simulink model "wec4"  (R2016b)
settings: Solver=ode4  StartTime=0  StopTime=1000  FixedStep=0.005  MaxStep=0.005  RelTol=1e-3  EnableMultiTasking=on
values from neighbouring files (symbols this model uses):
  arAdaptiveLawData = 1/2*zModelSimple.zModelPto.arFreq.*     zModelSimple.zModelPto.arMagnitude./     cos(zModelSimple.zModelPto.arPhase*pi/180+pi/2)    [IMPACT_Control.m]
  arAdaptiveLawDataX = 1/2*zModelSimpleX.zModelPto.arFreq.*         zModelSimpleX.zModelPto.arMagnitude./         cos(zModelSimpleX.zModelPto.arPhase*pi/180+pi/2)    [IMPACT_Control.m]
  arControllerRampGain = [0,0,1,1]    [IMPACT_Control.m]
  arControllerRampTime = [0 rStartRampTime rStartRampTime+rRampTimeLength 8000]    [IMPACT_Control.m]
  arEkfInitialisation = zeros(1,11)    [IMPACT_Control.m]
  arEkfInitialisationX = zeros(1,11)    [IMPACT_Control.m]
  arFrequency = zModelSimple.zModelPto.arFreq    [IMPACT_Control.m]
  arFrequencyRange = zModelSimple.zModelPto.arFreq    [IMPACT_Control.m]
  arFrequencyX = zModelSimpleX.zModelPto.arFreq    [IMPACT_Control.m]
  arImpedance = 1./zModelSimple.zModelPto.arMagnitude./zModelSimple.zModelPto.arFreq    [IMPACT_Control.m]
  arImpedanceX = 1./zModelSimpleX.zModelPto.arMagnitude./zModelSimpleX.zModelPto.arFreq    [IMPACT_Control.m]
  CentralPTOPreload = -1.6113e+07    (= -16113000)    [wecSimInputFile.m]
  F1 = [4.243 2.375 -12.243]    [wecSimInputFile.m]
  F2 = [4.243 -2.375 -12.243]    [wecSimInputFile.m]
  F3 = [-4.243 -2.375 -12.243]    [wecSimInputFile.m]
  F4 = [-4.243 2.375 -12.243]    [wecSimInputFile.m]
  FC = [0 0 -14]    [wecSimInputFile.m]
  iAdaptiveDamping = 0    [wec4IMPACT_Project.m]    (also in IMPACT_Control.m = handles.iAdaptiveDamping; wec1_IMPACT_Project.m; wec2_IMPACT_Project.m; wec3_IMPACT_Project.m)
  iControlType = 2    [wec4IMPACT_Project.m]    (also in IMPACT_Control.m = handles.iControlType; wec1_IMPACT_Project.m = 1; wec2_IMPACT_Project.m = 1; wec3_IMPACT_Project.m = 1)
  iPtoPositionConstraint = 1    [wec4IMPACT_Project.m]    (also in IMPACT_Control.m = handles.iPtoPositionConstraint; wec1_IMPACT_Project.m = 0; wec2_IMPACT_Project.m; wec3_IMPACT_Project.m)
  iSensorNoise = 0    [IMPACT_Control.m]
  m = m+1    (= 2)    [checkParamFile.m]
  PTOrotation = atan((T1(2)-F1(2))/(T1(1)-F1(1)))    [wecSimInputFile.m]
  rCogFloater = -8    [wec4_IMPACT_Model.m]    (also in paramInitial.m = get( handles.edit_rCogFloater, 'String' ); wec1_IMPACT_Model.m = -18; wec2_IMPACT_Model.m = -8.5; wec3_IMPACT_Model.m = -0.7)
  rCogSpar = -36.6    [wec4_IMPACT_Model.m]    (also in paramInitial.m = get( handles.edit_rCogSpar, 'String' ); wec3_IMPACT_Model.m = -21.3; wec3_IMPACT_Model2.m = -21.3)
  rDisplacementLimit = 10.000000    (= 10)    [wec4IMPACT_Project.m]    (also in IMPACT_Control.m = getValue(handles.edit_displacementLimit); wec1_IMPACT_Project.m; wec2_IMPACT_Project.m; wec3_IMPACT_Project.m = 3)
  rDisplacementLimitX = 10.000000    (= 10)    [wec4IMPACT_Project.m]    (also in IMPACT_Control.m = getValue(handles.edit_displacementLimitX); wec1_IMPACT_Project.m = 0; wec2_IMPACT_Project.m; wec3_IMPACT_Project.m = 0)
  rGainForAntiWIndUp = tfControllerDiscrete.rGain    [IMPACT_Control.m]
  rGainForAntiWIndUpX = tfControllerXDiscrete.rGain    [IMPACT_Control.m]
  rMaxForcePto = 300000000.000000    (= 300000000)    [wec4IMPACT_Project.m]    (also in IMPACT_Control.m = getValue(handles.edit_maxForcePto); wec1_IMPACT_Project.m = 1e+15; wec2_IMPACT_Project.m = 1e+15; wec3_IMPACT_Project.m = 1000000000)
  rMinForcePto = -300000000.000000    (= -300000000)    [wec4IMPACT_Project.m]    (also in IMPACT_Control.m = getValue(handles.edit_minForcePto); wec1_IMPACT_Project.m = -1e+15; wec2_IMPACT_Project.m = -1e+15; wec3_IMPACT_Project.m = -1000000000)
  rMooringX = 20000    [wec4_IMPACT_Model.m]    (also in paramInitial.m = get( handles.edit_rMooringX, 'String' ); wec3_IMPACT_Model.m = 10000; wec3_IMPACT_Model2.m = 10000)
  rMooringZ = 10000    [wec4_IMPACT_Model.m]    (also in paramInitial.m = get( handles.edit_rMooringZ, 'String' ); wec3_IMPACT_Model.m = 0; wec3_IMPACT_Model2.m = 0)
  rOutputSampleTime = 0.010000    (= 0.01)    [wec4IMPACT_Project.m]    (also in IMPACT_Control.m = getValue(handles.edit_outputSampleTime); wec1_IMPACT_Project.m; wec2_IMPACT_Project.m; wec3_IMPACT_Project.m)
  rPassiveDampingGain = -604830.000000    (= -604830)    [wec4IMPACT_Project.m]    (also in IMPACT_Control.m = getValue(handles.edit_gainPLD); wec1_IMPACT_Project.m = -214018.1537; wec2_IMPACT_Project.m = -1948070; wec3_IMPACT_Project.m = -519390)
  rPassiveDampingGainX = -278660.000000    (= -278660)    [wec4IMPACT_Project.m]    (also in IMPACT_Control.m = getValue(handles.edit_gainPLDX); wec1_IMPACT_Project.m = 0; wec2_IMPACT_Project.m = 0; wec3_IMPACT_Project.m = 0)
  rTetherPretension = 1.6113e+07    (= 16113000)    [wec4_IMPACT_Model.m]    (also in paramInitial.m = get( handles.edit_rTetherPretension, 'String' ); wec3_IMPACT_Model.m = 0; wec3_IMPACT_Model2.m = 0)
  rTetherSpring = 500000    [wec4_IMPACT_Model.m]    (also in paramInitial.m = get( handles.edit_rTetherSpring, 'String' ); wec3_IMPACT_Model.m = 0; wec3_IMPACT_Model2.m = 0)
  rUpperFrequencyLimit = EKFFloater.upperFreq    [IMPACT_Control.m]
  rXf = 4.243    [wec4AdditionalParams.m]
  rXs = 16.075    [wec4AdditionalParams.m]
  rYf = 2.375    [wec4AdditionalParams.m]
  rYs = 16.075    [wec4AdditionalParams.m]
  rZf = 4.243    [wec4AdditionalParams.m]
  rZs = 2.4350    (= 2.435)    [wec4AdditionalParams.m]
  rZTetherF = 6    [wec4AdditionalParams.m]
  rZTetherS = 2.4350    (= 2.435)    [wec4AdditionalParams.m]
  s = tf('s')    [wec4_IMPACT_Model.m]    (also in IMPACT_Control.m; wec1_IMPACT_Model.m; wec2_IMPACT_Model.m; wec3_IMPACT_Model.m)
  SidePTO1Preload = PreloadPTOCorner    (= 0)    [wecSimInputFile.m]
  SidePTO2Preload = PreloadPTOCorner    (= 0)    [wecSimInputFile.m]
  SidePTO3Preload = PreloadPTOCorner    (= 0)    [wecSimInputFile.m]
  SidePTO4Preload = PreloadPTOCorner    (= 0)    [wecSimInputFile.m]
  simu = simulationClass()    [wecSimInputFile.m]
  T1 = [16.075 16.075 -34.165]    [wecSimInputFile.m]
  T2 = [16.075 -16.075 -34.165]    [wecSimInputFile.m]
  T3 = [-16.075 -16.075 -34.165]    [wecSimInputFile.m]
  T4 = [-16.075 16.075 -34.165]    [wecSimInputFile.m]
  TC = [0 0 -34.165]    [wecSimInputFile.m]
  waves = waveClass('irregular')    [wecSimInputFile.m]
  Z = magPhaseToComplex(zModelTf)    [IMPACT_Control.m]
undefined symbols (not defined in the file or in its folder): arControllerDiscreteDen, arControllerDiscreteNum, arControllerDiscreteXDen, arControllerDiscreteXNum, arExcForceFloaterDen, arExcForceFloaterNum, arExcForceFloaterXDen, arExcForceFloaterXNum, arExcForceSparDen, arExcForceSparNum, arExcForceSparXDen, arExcForceSparXNum, arFexcFloaterDen, arFexcFloaterNum, arFexcFloaterXDen, arFexcFloaterXNum, arFexcSparDen, arFexcSparNum, arFexcSparXDen, arFexcSparXNum, Body, body, constraint, CTTime, deg, Elements, geometry, IRKB, kg, lenJ, mooring, N, pto, rAccelerationGainFloater, rAccelerationGainFloaterX, rAccelerationGainSpar, rAccelerationGainSparX, rad, rBuoyancyGainFloater, rBuoyancyGainFloaterX, rBuoyancyGainSpar, rBuoyancyGainSparX, rDampingGainFloater, rDampingGainFloaterX, rDampingGainSpar, rDampingGainSparX, Rigid, rMaxFocePto, wec4_float, wec4_reactor, WECSim_Lib, X, Y
libraries: nesl_utility x380, sm_lib x170, vrlib x91, simulink x12, WECSim_Lib x4
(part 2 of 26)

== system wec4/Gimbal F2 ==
  Assignment : Assignment  DiagnosticForDimensions=Warning  IndexOptions=Index vector (dialog)  Indices=[4 5 6]  OutputSizes=1
  Assignment1 : Assignment  DiagnosticForDimensions=Warning  IndexOptions=Index vector (dialog)  Indices=[4 5 6]  OutputSizes=1
  Assignment2 : Assignment  DiagnosticForDimensions=Warning  IndexOptions=Index vector (dialog)  Indices=[4 5 6]  OutputSizes=1
  Assignment3 : Assignment  DiagnosticForDimensions=Warning  IndexOptions=Index vector (dialog)  Indices=2  OutputSizes=1
  Assignment4 : Assignment  DiagnosticForDimensions=Warning  IndexOptions=Index vector (dialog)  Indices=2  OutputSizes=1
  CONSTRAINT (Gimbal Joint) : sm_lib/Joints/Gimbal Joint  SenseConstraintForce=on  SenseConstraintForceX=off  SenseConstraintForceY=off  SenseConstraintForceZ=off  SenseConstraintTorque=on  SenseConstraintTorqueX=off  SenseConstraintTorqueY=off  SenseConstraintTorqueZ=off  SenseTotalForce=off  SenseTotalForceX=off  SenseTotalForceY=off  SenseTotalForceZ=off  SenseTotalTorque=off  SenseTotalTorqueX=off  SenseTotalTorqueY=off  SenseTotalTorqueZ=off  CompositeWrenchDir=BaseOnFollower  CompositeWrenchFrame=BaseFrame  RxEquilibriumPosition=0  RxEquilibriumPositionUnits=rad  RxSpringStiffness=top_const_k  RxSpringStiffnessUnits=N*m/rad  RxDampingCoefficient=top_const_c  RxDampingCoefficientUnits=N*m/(rad/s)  RxTorqueActuationMode=NoTorque  RxMotionActuationMode=ComputedMotion  RxSensePosition=on  RxSenseVelocity=on  RxSenseAcceleration=on  RxSenseTorqueForce=off  RxPositionTargetSpecify=off  RxPositionTargetPriority=High  RxPositionTargetValue=0  RxPositionTargetValueUnits=deg  RxVelocityTargetSpecify=off  RxVelocityTargetPriority=High  RxVelocityTargetValue=0  RxVelocityTargetValueUnits=deg/s  RyEquilibriumPosition=0  RyEquilibriumPositionUnits=rad  RySpringStiffness=top_const_k  RySpringStiffnessUnits=N*m/rad  RyDampingCoefficient=top_const_c  RyDampingCoefficientUnits=N*m/(rad/s)  RyTorqueActuationMode=NoTorque  RyMotionActuationMode=ComputedMotion  RySensePosition=on  RySenseVelocity=on  RySenseAcceleration=on  RySenseTorqueForce=off  RyPositionTargetSpecify=off  RyPositionTargetPriority=High  RyPositionTargetValue=0  RyPositionTargetValueUnits=deg  RyVelocityTargetSpecify=off  RyVelocityTargetPriority=High  RyVelocityTargetValue=0  RyVelocityTargetValueUnits=deg/s  RzEquilibriumPosition=0  RzEquilibriumPositionUnits=rad  RzSpringStiffness=top_const_k  RzSpringStiffnessUnits=N*m/rad  RzDampingCoefficient=top_const_c  RzDampingCoefficientUnits=N*m/(rad/s)  RzTorqueActuationMode=NoTorque  RzMotionActuationMode=ComputedMotion  RzSensePosition=on  RzSenseVelocity=on  RzSenseAcceleration=on  RzSenseTorqueForce=off  RzPositionTargetSpecify=off  RzPositionTargetPriority=High  RzPositionTargetValue=0  RzPositionTargetValueUnits=deg  RzVelocityTargetSpecify=off  RzVelocityTargetPriority=High  RzVelocityTargetValue=0  RzVelocityTargetValueUnits=deg/s
  Constant : Constant  Value=[0 0 0 0 0 0]
  Constant1 : Constant  Value=[0 0 0 0 0 0]
  Constant2 : Constant  Value=[0 0 0 0 0 0]
  Gain{1..5} (5 alike) : Gain  Gain=-1
  Mux : Mux  Inputs=2
  Mux1 : Mux
  Mux2 : Mux  Inputs=3
  Mux3 : Mux  Inputs=3
  Mux4 : Mux  Inputs=3
  PS-Simulink Converter{1..11} (11 alike) : nesl_utility/PS-Simulink Converter  PhysicalDomain=network_engine_domain  SubClassName=ps_output  LeftPortType=input  RightPortType=output  PseudoPeriodic=off  Frequencies=[]  Unit=1  AffineConversion=off
  Rigid Transform (Position) : sm_lib/Frames and Transforms/Rigid Transform  TranslationMethod=Cartesian  TranslationStandardOffset=0  TranslationLengthUnit=m  TranslationStandardAxis=+Z  TranslationCartesianOffset=constraint.initDisp.initLinDisp+constraint.loc  TranslationROffset=0  TranslationROffsetUnits=m  TranslationZOffset=0  TranslationZOffsetUnits=m  TranslationThetaOffset=0  TranslationThetaOffsetUnits=deg  RotationMethod=None  RotationAngleUnits=rad  RotationStandardAxis=+Y  RotationAngle=0  RotationArbitraryAxis=[0 1 0]  FollAlignAxisA=+X  BaseAlignAxisA=+Y  FollAlignAxisB=+Y  BaseAlignAxisB=+Z  RotationSequenceAxes=FollowerAxes  RotationSequence=XYX  RotationSequenceAngles=[0 0 0]  RotationSequenceAnglesUnits=deg  RotationMatrix=[1 0 0; 0 1 0; 0 0 1]
  Rigid Transform (Position)1 : sm_lib/Frames and Transforms/Rigid Transform  TranslationMethod=Cartesian  TranslationStandardOffset=0  TranslationLengthUnit=m  TranslationStandardAxis=+Z  TranslationCartesianOffset=constraint.initDisp.initLinDisp+constraint.loc  TranslationROffset=0  TranslationROffsetUnits=m  TranslationZOffset=0  TranslationZOffsetUnits=m  TranslationThetaOffset=0  TranslationThetaOffsetUnits=deg  RotationMethod=None  RotationAngleUnits=rad  RotationStandardAxis=+Y  RotationAngle=0  RotationArbitraryAxis=[0 1 0]  FollAlignAxisA=+X  BaseAlignAxisA=+Y  FollAlignAxisB=+Y  BaseAlignAxisB=+Z  RotationSequenceAxes=FollowerAxes  RotationSequence=XYX  RotationSequenceAngles=[0 0 0]  RotationSequenceAnglesUnits=deg  RotationMatrix=[1 0 0; 0 1 0; 0 0 1]
  Rigid Transform (90 X) : sm_lib/Frames and Transforms/Rigid Transform  TranslationMethod=None  TranslationStandardOffset=0  TranslationLengthUnit=m  TranslationStandardAxis=+Z  TranslationCartesianOffset=constraint.loc  TranslationROffset=0  TranslationROffsetUnits=m  TranslationZOffset=0  TranslationZOffsetUnits=m  TranslationThetaOffset=0  TranslationThetaOffsetUnits=deg  RotationMethod=StandardAxis  RotationAngleUnits=deg  RotationStandardAxis=+X  RotationAngle=90  RotationArbitraryAxis=[0 1 0]  FollAlignAxisA=+X  BaseAlignAxisA=+Y  FollAlignAxisB=+Y  BaseAlignAxisB=+Z  RotationSequenceAxes=FollowerAxes  RotationSequence=XYX  RotationSequenceAngles=[0 0 0]  RotationSequenceAnglesUnits=deg  RotationMatrix=[1 0 0; 0 1 0; 0 0 1]
  Rigid Transform (90 X)1 : sm_lib/Frames and Transforms/Rigid Transform  TranslationMethod=None  TranslationStandardOffset=0  TranslationLengthUnit=m  TranslationStandardAxis=+Z  TranslationCartesianOffset=constraint.loc  TranslationROffset=0  TranslationROffsetUnits=m  TranslationZOffset=0  TranslationZOffsetUnits=m  TranslationThetaOffset=0  TranslationThetaOffsetUnits=deg  RotationMethod=StandardAxis  RotationAngleUnits=deg  RotationStandardAxis=+X  RotationAngle=90  RotationArbitraryAxis=[0 1 0]  FollAlignAxisA=+X  BaseAlignAxisA=+Y  FollAlignAxisB=+Y  BaseAlignAxisB=+Z  RotationSequenceAxes=FollowerAxes  RotationSequence=XYX  RotationSequenceAngles=[0 0 0]  RotationSequenceAnglesUnits=deg  RotationMatrix=[1 0 0; 0 1 0; 0 0 1]
  Rigid Transform (Orientation) : sm_lib/Frames and Transforms/Rigid Transform  TranslationMethod=None  TranslationStandardOffset=0  TranslationLengthUnit=m  TranslationStandardAxis=+Z  TranslationCartesianOffset=constraint.loc  TranslationROffset=0  TranslationROffsetUnits=m  TranslationZOffset=0  TranslationZOffsetUnits=m  TranslationThetaOffset=0  TranslationThetaOffsetUnits=deg  RotationMethod=RotationMatrix  RotationAngleUnits=rad  RotationStandardAxis=+Y  RotationAngle=0  RotationArbitraryAxis=[0 1 0]  FollAlignAxisA=+X  BaseAlignAxisA=+Y  FollAlignAxisB=+Y  BaseAlignAxisB=+Z  RotationSequenceAxes=FollowerAxes  RotationSequence=XYX  RotationSequenceAngles=[0 0 0]  RotationSequenceAnglesUnits=deg  RotationMatrix=constraint.orientation.rotationMatrix
  Rigid Transform (Orientation)1 : sm_lib/Frames and Transforms/Rigid Transform  TranslationMethod=None  TranslationStandardOffset=0  TranslationLengthUnit=m  TranslationStandardAxis=+Z  TranslationCartesianOffset=constraint.loc  TranslationROffset=0  TranslationROffsetUnits=m  TranslationZOffset=0  TranslationZOffsetUnits=m  TranslationThetaOffset=0  TranslationThetaOffsetUnits=deg  RotationMethod=RotationMatrix  RotationAngleUnits=rad  RotationStandardAxis=+Y  RotationAngle=0  RotationArbitraryAxis=[0 1 0]  FollAlignAxisA=+X  BaseAlignAxisA=+Y  FollAlignAxisB=+Y  BaseAlignAxisB=+Z  RotationSequenceAxes=FollowerAxes  RotationSequence=XYX  RotationSequenceAngles=[0 0 0]  RotationSequenceAnglesUnits=deg  RotationMatrix=constraint.orientation.rotationMatrix
  Selector : Selector  InputPortWidth=3  IndexOptions=Index vector (dialog)  Indices=[1 3 2]  OutputSizes=1
  Selector1 : Selector  InputPortWidth=3  IndexOptions=Index vector (dialog)  Indices=[2]  OutputSizes=1
  Selector2 : Selector  InputPortWidth=3  IndexOptions=Index vector (dialog)  Indices=[1 3 2]  OutputSizes=1
  Selector3 : Selector  InputPortWidth=3  IndexOptions=Index vector (dialog)  Indices=[2]  OutputSizes=1
  output : ToWorkspace  VariableName=constraint7_out  SaveFormat=Structure With Time  SampleTime=-1
  F : PMIOPort  Port=1  Side=Right
  B : PMIOPort  Port=2  Side=Left
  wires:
  Assignment4/1 -> Mux/2
  PS-Simulink Converter4/1 -> Selector2/1
  Gain4/1 -> Assignment4/2
  Selector3/1 -> Gain4/1
  Selector2/1 -> Assignment4/1, Selector3/1
  Assignment3/1 -> Mux/1
  Gain3/1 -> Assignment3/2
  Selector1/1 -> Gain3/1
  Selector/1 -> Selector1/1, Assignment3/1
  PS-Simulink Converter3/1 -> Selector/1
  Mux3/1 -> Assignment1/2
  Mux4/1 -> Assignment/2
  Constant/1 -> Assignment/1
  Constant1/1 -> Assignment1/1
  Constant2/1 -> Assignment2/1
  Assignment2/1 -> Mux1/3  "acceleration"
  Assignment1/1 -> Mux1/2  "velocity"
  Assignment/1 -> Mux1/1  "position"
  Mux/1 -> Mux1/4  "Constraint Forces"
  Mux1/1 -> output/1
  PS-Simulink Converter5/1 -> Gain5/1
  Gain5/1 -> Mux2/2
  PS-Simulink Converter6/1 -> Mux2/3
  PS-Simulink Converter7/1 -> Mux2/1
  Mux2/1 -> Assignment2/2
  PS-Simulink Converter2/1 -> Gain2/1
  Gain2/1 -> Mux3/2
  PS-Simulink Converter8/1 -> Mux3/3
  PS-Simulink Converter9/1 -> Mux3/1
  PS-Simulink Converter11/1 -> Gain1/1
  Gain1/1 -> Mux4/2
  PS-Simulink Converter1/1 -> Mux4/1
  PS-Simulink Converter10/1 -> Mux4/3
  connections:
  Rigid Transform (Position)1/LConn1 -- F/RConn1
  Rigid Transform (Position)1/RConn1 -- Rigid Transform (Orientation)1/LConn1
  Rigid Transform (Orientation)1/RConn1 -- Rigid Transform (90 X)1/LConn1
  Rigid Transform (Orientation)/RConn1 -- Rigid Transform (90 X)/LConn1
  Rigid Transform (Position)/RConn1 -- Rigid Transform (Orientation)/LConn1
  Rigid Transform (Position)/LConn1 -- B/RConn1
  PS-Simulink Converter4/LConn1 -- CONSTRAINT (Gimbal Joint)/RConn12
  PS-Simulink Converter3/LConn1 -- CONSTRAINT (Gimbal Joint)/RConn11
  PS-Simulink Converter5/LConn1 -- CONSTRAINT (Gimbal Joint)/RConn10
  PS-Simulink Converter6/LConn1 -- CONSTRAINT (Gimbal Joint)/RConn7
  PS-Simulink Converter7/LConn1 -- CONSTRAINT (Gimbal Joint)/RConn4
  CONSTRAINT (Gimbal Joint)/LConn1 -- Rigid Transform (90 X)/RConn1
  PS-Simulink Converter2/LConn1 -- CONSTRAINT (Gimbal Joint)/RConn9
  CONSTRAINT (Gimbal Joint)/RConn6 -- PS-Simulink Converter8/LConn1
  PS-Simulink Converter9/LConn1 -- CONSTRAINT (Gimbal Joint)/RConn3
  CONSTRAINT (Gimbal Joint)/RConn2 -- PS-Simulink Converter1/LConn1
  CONSTRAINT (Gimbal Joint)/RConn5 -- PS-Simulink Converter10/LConn1
  PS-Simulink Converter11/LConn1 -- CONSTRAINT (Gimbal Joint)/RConn8
  Rigid Transform (90 X)1/RConn1 -- CONSTRAINT (Gimbal Joint)/RConn1

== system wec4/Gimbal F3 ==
  Assignment : Assignment  DiagnosticForDimensions=Warning  IndexOptions=Index vector (dialog)  Indices=[4 5 6]  OutputSizes=1
  Assignment1 : Assignment  DiagnosticForDimensions=Warning  IndexOptions=Index vector (dialog)  Indices=[4 5 6]  OutputSizes=1
  Assignment2 : Assignment  DiagnosticForDimensions=Warning  IndexOptions=Index vector (dialog)  Indices=[4 5 6]  OutputSizes=1
  Assignment3 : Assignment  DiagnosticForDimensions=Warning  IndexOptions=Index vector (dialog)  Indices=2  OutputSizes=1
  Assignment4 : Assignment  DiagnosticForDimensions=Warning  IndexOptions=Index vector (dialog)  Indices=2  OutputSizes=1
  CONSTRAINT (Gimbal Joint) : sm_lib/Joints/Gimbal Joint  SenseConstraintForce=on  SenseConstraintForceX=off  SenseConstraintForceY=off  SenseConstraintForceZ=off  SenseConstraintTorque=on  SenseConstraintTorqueX=off  SenseConstraintTorqueY=off  SenseConstraintTorqueZ=off  SenseTotalForce=off  SenseTotalForceX=off  SenseTotalForceY=off  SenseTotalForceZ=off  SenseTotalTorque=off  SenseTotalTorqueX=off  SenseTotalTorqueY=off  SenseTotalTorqueZ=off  CompositeWrenchDir=BaseOnFollower  CompositeWrenchFrame=BaseFrame  RxEquilibriumPosition=0  RxEquilibriumPositionUnits=rad  RxSpringStiffness=top_const_k  RxSpringStiffnessUnits=N*m/rad  RxDampingCoefficient=top_const_c  RxDampingCoefficientUnits=N*m/(rad/s)  RxTorqueActuationMode=NoTorque  RxMotionActuationMode=ComputedMotion  RxSensePosition=on  RxSenseVelocity=on  RxSenseAcceleration=on  RxSenseTorqueForce=off  RxPositionTargetSpecify=off  RxPositionTargetPriority=High  RxPositionTargetValue=0  RxPositionTargetValueUnits=deg  RxVelocityTargetSpecify=off  RxVelocityTargetPriority=High  RxVelocityTargetValue=0  RxVelocityTargetValueUnits=deg/s  RyEquilibriumPosition=0  RyEquilibriumPositionUnits=rad  RySpringStiffness=top_const_k  RySpringStiffnessUnits=N*m/rad  RyDampingCoefficient=top_const_c  RyDampingCoefficientUnits=N*m/(rad/s)  RyTorqueActuationMode=NoTorque  RyMotionActuationMode=ComputedMotion  RySensePosition=on  RySenseVelocity=on  RySenseAcceleration=on  RySenseTorqueForce=off  RyPositionTargetSpecify=off  RyPositionTargetPriority=High  RyPositionTargetValue=0  RyPositionTargetValueUnits=deg  RyVelocityTargetSpecify=off  RyVelocityTargetPriority=High  RyVelocityTargetValue=0  RyVelocityTargetValueUnits=deg/s  RzEquilibriumPosition=0  RzEquilibriumPositionUnits=rad  RzSpringStiffness=top_const_k  RzSpringStiffnessUnits=N*m/rad  RzDampingCoefficient=top_const_c  RzDampingCoefficientUnits=N*m/(rad/s)  RzTorqueActuationMode=NoTorque  RzMotionActuationMode=ComputedMotion  RzSensePosition=on  RzSenseVelocity=on  RzSenseAcceleration=on  RzSenseTorqueForce=off  RzPositionTargetSpecify=off  RzPositionTargetPriority=High  RzPositionTargetValue=0  RzPositionTargetValueUnits=deg  RzVelocityTargetSpecify=off  RzVelocityTargetPriority=High  RzVelocityTargetValue=0  RzVelocityTargetValueUnits=deg/s
  Constant : Constant  Value=[0 0 0 0 0 0]
  Constant1 : Constant  Value=[0 0 0 0 0 0]
  Constant2 : Constant  Value=[0 0 0 0 0 0]
  Gain{1..5} (5 alike) : Gain  Gain=-1
  Mux : Mux  Inputs=2
  Mux1 : Mux
  Mux2 : Mux  Inputs=3
  Mux3 : Mux  Inputs=3
  Mux4 : Mux  Inputs=3
  PS-Simulink Converter{1..11} (11 alike) : nesl_utility/PS-Simulink Converter  PhysicalDomain=network_engine_domain  SubClassName=ps_output  LeftPortType=input  RightPortType=output  PseudoPeriodic=off  Frequencies=[]  Unit=1  AffineConversion=off
  Rigid Transform (Position) : sm_lib/Frames and Transforms/Rigid Transform  TranslationMethod=Cartesian  TranslationStandardOffset=0  TranslationLengthUnit=m  TranslationStandardAxis=+Z  TranslationCartesianOffset=constraint.initDisp.initLinDisp+constraint.loc  TranslationROffset=0  TranslationROffsetUnits=m  TranslationZOffset=0  TranslationZOffsetUnits=m  TranslationThetaOffset=0  TranslationThetaOffsetUnits=deg  RotationMethod=None  RotationAngleUnits=rad  RotationStandardAxis=+Y  RotationAngle=0  RotationArbitraryAxis=[0 1 0]  FollAlignAxisA=+X  BaseAlignAxisA=+Y  FollAlignAxisB=+Y  BaseAlignAxisB=+Z  RotationSequenceAxes=FollowerAxes  RotationSequence=XYX  RotationSequenceAngles=[0 0 0]  RotationSequenceAnglesUnits=deg  RotationMatrix=[1 0 0; 0 1 0; 0 0 1]
  Rigid Transform (Position)1 : sm_lib/Frames and Transforms/Rigid Transform  TranslationMethod=Cartesian  TranslationStandardOffset=0  TranslationLengthUnit=m  TranslationStandardAxis=+Z  TranslationCartesianOffset=constraint.initDisp.initLinDisp+constraint.loc  TranslationROffset=0  TranslationROffsetUnits=m  TranslationZOffset=0  TranslationZOffsetUnits=m  TranslationThetaOffset=0  TranslationThetaOffsetUnits=deg  RotationMethod=None  RotationAngleUnits=rad  RotationStandardAxis=+Y  RotationAngle=0  RotationArbitraryAxis=[0 1 0]  FollAlignAxisA=+X  BaseAlignAxisA=+Y  FollAlignAxisB=+Y  BaseAlignAxisB=+Z  RotationSequenceAxes=FollowerAxes  RotationSequence=XYX  RotationSequenceAngles=[0 0 0]  RotationSequenceAnglesUnits=deg  RotationMatrix=[1 0 0; 0 1 0; 0 0 1]
  Rigid Transform (90 X) : sm_lib/Frames and Transforms/Rigid Transform  TranslationMethod=None  TranslationStandardOffset=0  TranslationLengthUnit=m  TranslationStandardAxis=+Z  TranslationCartesianOffset=constraint.loc  TranslationROffset=0  TranslationROffsetUnits=m  TranslationZOffset=0  TranslationZOffsetUnits=m  TranslationThetaOffset=0  TranslationThetaOffsetUnits=deg  RotationMethod=StandardAxis  RotationAngleUnits=deg  RotationStandardAxis=+X  RotationAngle=90  RotationArbitraryAxis=[0 1 0]  FollAlignAxisA=+X  BaseAlignAxisA=+Y  FollAlignAxisB=+Y  BaseAlignAxisB=+Z  RotationSequenceAxes=FollowerAxes  RotationSequence=XYX  RotationSequenceAngles=[0 0 0]  RotationSequenceAnglesUnits=deg  RotationMatrix=[1 0 0; 0 1 0; 0 0 1]
  Rigid Transform (90 X)1 : sm_lib/Frames and Transforms/Rigid Transform  TranslationMethod=None  TranslationStandardOffset=0  TranslationLengthUnit=m  TranslationStandardAxis=+Z  TranslationCartesianOffset=constraint.loc  TranslationROffset=0  TranslationROffsetUnits=m  TranslationZOffset=0  TranslationZOffsetUnits=m  TranslationThetaOffset=0  TranslationThetaOffsetUnits=deg  RotationMethod=StandardAxis  RotationAngleUnits=deg  RotationStandardAxis=+X  RotationAngle=90  RotationArbitraryAxis=[0 1 0]  FollAlignAxisA=+X  BaseAlignAxisA=+Y  FollAlignAxisB=+Y  BaseAlignAxisB=+Z  RotationSequenceAxes=FollowerAxes  RotationSequence=XYX  RotationSequenceAngles=[0 0 0]  RotationSequenceAnglesUnits=deg  RotationMatrix=[1 0 0; 0 1 0; 0 0 1]
  Rigid Transform (Orientation) : sm_lib/Frames and Transforms/Rigid Transform  TranslationMethod=None  TranslationStandardOffset=0  TranslationLengthUnit=m  TranslationStandardAxis=+Z  TranslationCartesianOffset=constraint.loc  TranslationROffset=0  TranslationROffsetUnits=m  TranslationZOffset=0  TranslationZOffsetUnits=m  TranslationThetaOffset=0  TranslationThetaOffsetUnits=deg  RotationMethod=RotationMatrix  RotationAngleUnits=rad  RotationStandardAxis=+Y  RotationAngle=0  RotationArbitraryAxis=[0 1 0]  FollAlignAxisA=+X  BaseAlignAxisA=+Y  FollAlignAxisB=+Y  BaseAlignAxisB=+Z  RotationSequenceAxes=FollowerAxes  RotationSequence=XYX  RotationSequenceAngles=[0 0 0]  RotationSequenceAnglesUnits=deg  RotationMatrix=constraint.orientation.rotationMatrix
  Rigid Transform (Orientation)1 : sm_lib/Frames and Transforms/Rigid Transform  TranslationMethod=None  TranslationStandardOffset=0  TranslationLengthUnit=m  TranslationStandardAxis=+Z  TranslationCartesianOffset=constraint.loc  TranslationROffset=0  TranslationROffsetUnits=m  TranslationZOffset=0  TranslationZOffsetUnits=m  TranslationThetaOffset=0  TranslationThetaOffsetUnits=deg  RotationMethod=RotationMatrix  RotationAngleUnits=rad  RotationStandardAxis=+Y  RotationAngle=0  RotationArbitraryAxis=[0 1 0]  FollAlignAxisA=+X  BaseAlignAxisA=+Y  FollAlignAxisB=+Y  BaseAlignAxisB=+Z  RotationSequenceAxes=FollowerAxes  RotationSequence=XYX  RotationSequenceAngles=[0 0 0]  RotationSequenceAnglesUnits=deg  RotationMatrix=constraint.orientation.rotationMatrix
  Selector : Selector  InputPortWidth=3  IndexOptions=Index vector (dialog)  Indices=[1 3 2]  OutputSizes=1
  Selector1 : Selector  InputPortWidth=3  IndexOptions=Index vector (dialog)  Indices=[2]  OutputSizes=1
  Selector2 : Selector  InputPortWidth=3  IndexOptions=Index vector (dialog)  Indices=[1 3 2]  OutputSizes=1
  Selector3 : Selector  InputPortWidth=3  IndexOptions=Index vector (dialog)  Indices=[2]  OutputSizes=1
  output : ToWorkspace  VariableName=constraint9_out  SaveFormat=Structure With Time  SampleTime=-1
  F : PMIOPort  Port=1  Side=Right
  B : PMIOPort  Port=2  Side=Left
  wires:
  Assignment4/1 -> Mux/2
  PS-Simulink Converter4/1 -> Selector2/1
  Gain4/1 -> Assignment4/2
  Selector3/1 -> Gain4/1
  Selector2/1 -> Assignment4/1, Selector3/1
  Assignment3/1 -> Mux/1
  Gain3/1 -> Assignment3/2
  Selector1/1 -> Gain3/1
  Selector/1 -> Selector1/1, Assignment3/1
  PS-Simulink Converter3/1 -> Selector/1
  Mux3/1 -> Assignment1/2
  Mux4/1 -> Assignment/2
  Constant/1 -> Assignment/1
  Constant1/1 -> Assignment1/1
  Constant2/1 -> Assignment2/1
  Assignment2/1 -> Mux1/3  "acceleration"
  Assignment1/1 -> Mux1/2  "velocity"
  Assignment/1 -> Mux1/1  "position"
  Mux/1 -> Mux1/4  "Constraint Forces"
  Mux1/1 -> output/1
  PS-Simulink Converter5/1 -> Gain5/1
  Gain5/1 -> Mux2/2
  PS-Simulink Converter6/1 -> Mux2/3
  PS-Simulink Converter7/1 -> Mux2/1
  Mux2/1 -> Assignment2/2
  PS-Simulink Converter2/1 -> Gain2/1
  Gain2/1 -> Mux3/2
  PS-Simulink Converter8/1 -> Mux3/3
  PS-Simulink Converter9/1 -> Mux3/1
  PS-Simulink Converter11/1 -> Gain1/1
  Gain1/1 -> Mux4/2
  PS-Simulink Converter1/1 -> Mux4/1
  PS-Simulink Converter10/1 -> Mux4/3
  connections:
  Rigid Transform (Position)1/LConn1 -- F/RConn1
  Rigid Transform (Position)1/RConn1 -- Rigid Transform (Orientation)1/LConn1
  Rigid Transform (Orientation)1/RConn1 -- Rigid Transform (90 X)1/LConn1
  Rigid Transform (Orientation)/RConn1 -- Rigid Transform (90 X)/LConn1
  Rigid Transform (Position)/RConn1 -- Rigid Transform (Orientation)/LConn1
  Rigid Transform (Position)/LConn1 -- B/RConn1
  PS-Simulink Converter4/LConn1 -- CONSTRAINT (Gimbal Joint)/RConn12
  PS-Simulink Converter3/LConn1 -- CONSTRAINT (Gimbal Joint)/RConn11
  PS-Simulink Converter5/LConn1 -- CONSTRAINT (Gimbal Joint)/RConn10
  PS-Simulink Converter6/LConn1 -- CONSTRAINT (Gimbal Joint)/RConn7
  PS-Simulink Converter7/LConn1 -- CONSTRAINT (Gimbal Joint)/RConn4
  CONSTRAINT (Gimbal Joint)/LConn1 -- Rigid Transform (90 X)/RConn1
  PS-Simulink Converter2/LConn1 -- CONSTRAINT (Gimbal Joint)/RConn9
  CONSTRAINT (Gimbal Joint)/RConn6 -- PS-Simulink Converter8/LConn1
  PS-Simulink Converter9/LConn1 -- CONSTRAINT (Gimbal Joint)/RConn3
  CONSTRAINT (Gimbal Joint)/RConn2 -- PS-Simulink Converter1/LConn1
  CONSTRAINT (Gimbal Joint)/RConn5 -- PS-Simulink Converter10/LConn1
  PS-Simulink Converter11/LConn1 -- CONSTRAINT (Gimbal Joint)/RConn8
  Rigid Transform (90 X)1/RConn1 -- CONSTRAINT (Gimbal Joint)/RConn1

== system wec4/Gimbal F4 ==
  Assignment : Assignment  DiagnosticForDimensions=Warning  IndexOptions=Index vector (dialog)  Indices=[4 5 6]  OutputSizes=1
  Assignment1 : Assignment  DiagnosticForDimensions=Warning  IndexOptions=Index vector (dialog)  Indices=[4 5 6]  OutputSizes=1
  Assignment2 : Assignment  DiagnosticForDimensions=Warning  IndexOptions=Index vector (dialog)  Indices=[4 5 6]  OutputSizes=1
  Assignment3 : Assignment  DiagnosticForDimensions=Warning  IndexOptions=Index vector (dialog)  Indices=2  OutputSizes=1
  Assignment4 : Assignment  DiagnosticForDimensions=Warning  IndexOptions=Index vector (dialog)  Indices=2  OutputSizes=1
  CONSTRAINT (Gimbal Joint) : sm_lib/Joints/Gimbal Joint  SenseConstraintForce=on  SenseConstraintForceX=off  SenseConstraintForceY=off  SenseConstraintForceZ=off  SenseConstraintTorque=on  SenseConstraintTorqueX=off  SenseConstraintTorqueY=off  SenseConstraintTorqueZ=off  SenseTotalForce=off  SenseTotalForceX=off  SenseTotalForceY=off  SenseTotalForceZ=off  SenseTotalTorque=off  SenseTotalTorqueX=off  SenseTotalTorqueY=off  SenseTotalTorqueZ=off  CompositeWrenchDir=BaseOnFollower  CompositeWrenchFrame=BaseFrame  RxEquilibriumPosition=0  RxEquilibriumPositionUnits=rad  RxSpringStiffness=top_const_k  RxSpringStiffnessUnits=N*m/rad  RxDampingCoefficient=top_const_c  RxDampingCoefficientUnits=N*m/(rad/s)  RxTorqueActuationMode=NoTorque  RxMotionActuationMode=ComputedMotion  RxSensePosition=on  RxSenseVelocity=on  RxSenseAcceleration=on  RxSenseTorqueForce=off  RxPositionTargetSpecify=off  RxPositionTargetPriority=High  RxPositionTargetValue=0  RxPositionTargetValueUnits=deg  RxVelocityTargetSpecify=off  RxVelocityTargetPriority=High  RxVelocityTargetValue=0  RxVelocityTargetValueUnits=deg/s  RyEquilibriumPosition=0  RyEquilibriumPositionUnits=rad  RySpringStiffness=top_const_k  RySpringStiffnessUnits=N*m/rad  RyDampingCoefficient=top_const_c  RyDampingCoefficientUnits=N*m/(rad/s)  RyTorqueActuationMode=NoTorque  RyMotionActuationMode=ComputedMotion  RySensePosition=on  RySenseVelocity=on  RySenseAcceleration=on  RySenseTorqueForce=off  RyPositionTargetSpecify=off  RyPositionTargetPriority=High  RyPositionTargetValue=0  RyPositionTargetValueUnits=deg  RyVelocityTargetSpecify=off  RyVelocityTargetPriority=High  RyVelocityTargetValue=0  RyVelocityTargetValueUnits=deg/s  RzEquilibriumPosition=0  RzEquilibriumPositionUnits=rad  RzSpringStiffness=top_const_k  RzSpringStiffnessUnits=N*m/rad  RzDampingCoefficient=top_const_c  RzDampingCoefficientUnits=N*m/(rad/s)  RzTorqueActuationMode=NoTorque  RzMotionActuationMode=ComputedMotion  RzSensePosition=on  RzSenseVelocity=on  RzSenseAcceleration=on  RzSenseTorqueForce=off  RzPositionTargetSpecify=off  RzPositionTargetPriority=High  RzPositionTargetValue=0  RzPositionTargetValueUnits=deg  RzVelocityTargetSpecify=off  RzVelocityTargetPriority=High  RzVelocityTargetValue=0  RzVelocityTargetValueUnits=deg/s
  Constant : Constant  Value=[0 0 0 0 0 0]
  Constant1 : Constant  Value=[0 0 0 0 0 0]
  Constant2 : Constant  Value=[0 0 0 0 0 0]
  Gain{1..5} (5 alike) : Gain  Gain=-1
  Mux : Mux  Inputs=2
  Mux1 : Mux
  Mux2 : Mux  Inputs=3
  Mux3 : Mux  Inputs=3
  Mux4 : Mux  Inputs=3
  PS-Simulink Converter{1..11} (11 alike) : nesl_utility/PS-Simulink Converter  PhysicalDomain=network_engine_domain  SubClassName=ps_output  LeftPortType=input  RightPortType=output  PseudoPeriodic=off  Frequencies=[]  Unit=1  AffineConversion=off
  Rigid Transform (Position) : sm_lib/Frames and Transforms/Rigid Transform  TranslationMethod=Cartesian  TranslationStandardOffset=0  TranslationLengthUnit=m  TranslationStandardAxis=+Z  TranslationCartesianOffset=constraint.initDisp.initLinDisp+constraint.loc  TranslationROffset=0  TranslationROffsetUnits=m  TranslationZOffset=0  TranslationZOffsetUnits=m  TranslationThetaOffset=0  TranslationThetaOffsetUnits=deg  RotationMethod=None  RotationAngleUnits=rad  RotationStandardAxis=+Y  RotationAngle=0  RotationArbitraryAxis=[0 1 0]  FollAlignAxisA=+X  BaseAlignAxisA=+Y  FollAlignAxisB=+Y  BaseAlignAxisB=+Z  RotationSequenceAxes=FollowerAxes  RotationSequence=XYX  RotationSequenceAngles=[0 0 0]  RotationSequenceAnglesUnits=deg  RotationMatrix=[1 0 0; 0 1 0; 0 0 1]
  Rigid Transform (Position)1 : sm_lib/Frames and Transforms/Rigid Transform  TranslationMethod=Cartesian  TranslationStandardOffset=0  TranslationLengthUnit=m  TranslationStandardAxis=+Z  TranslationCartesianOffset=constraint.initDisp.initLinDisp+constraint.loc  TranslationROffset=0  TranslationROffsetUnits=m  TranslationZOffset=0  TranslationZOffsetUnits=m  TranslationThetaOffset=0  TranslationThetaOffsetUnits=deg  RotationMethod=None  RotationAngleUnits=rad  RotationStandardAxis=+Y  RotationAngle=0  RotationArbitraryAxis=[0 1 0]  FollAlignAxisA=+X  BaseAlignAxisA=+Y  FollAlignAxisB=+Y  BaseAlignAxisB=+Z  RotationSequenceAxes=FollowerAxes  RotationSequence=XYX  RotationSequenceAngles=[0 0 0]  RotationSequenceAnglesUnits=deg  RotationMatrix=[1 0 0; 0 1 0; 0 0 1]
  Rigid Transform (90 X) : sm_lib/Frames and Transforms/Rigid Transform  TranslationMethod=None  TranslationStandardOffset=0  TranslationLengthUnit=m  TranslationStandardAxis=+Z  TranslationCartesianOffset=constraint.loc  TranslationROffset=0  TranslationROffsetUnits=m  TranslationZOffset=0  TranslationZOffsetUnits=m  TranslationThetaOffset=0  TranslationThetaOffsetUnits=deg  RotationMethod=StandardAxis  RotationAngleUnits=deg  RotationStandardAxis=+X  RotationAngle=90  RotationArbitraryAxis=[0 1 0]  FollAlignAxisA=+X  BaseAlignAxisA=+Y  FollAlignAxisB=+Y  BaseAlignAxisB=+Z  RotationSequenceAxes=FollowerAxes  RotationSequence=XYX  RotationSequenceAngles=[0 0 0]  RotationSequenceAnglesUnits=deg  RotationMatrix=[1 0 0; 0 1 0; 0 0 1]
  Rigid Transform (90 X)1 : sm_lib/Frames and Transforms/Rigid Transform  TranslationMethod=None  TranslationStandardOffset=0  TranslationLengthUnit=m  TranslationStandardAxis=+Z  TranslationCartesianOffset=constraint.loc  TranslationROffset=0  TranslationROffsetUnits=m  TranslationZOffset=0  TranslationZOffsetUnits=m  TranslationThetaOffset=0  TranslationThetaOffsetUnits=deg  RotationMethod=StandardAxis  RotationAngleUnits=deg  RotationStandardAxis=+X  RotationAngle=90  RotationArbitraryAxis=[0 1 0]  FollAlignAxisA=+X  BaseAlignAxisA=+Y  FollAlignAxisB=+Y  BaseAlignAxisB=+Z  RotationSequenceAxes=FollowerAxes  RotationSequence=XYX  RotationSequenceAngles=[0 0 0]  RotationSequenceAnglesUnits=deg  RotationMatrix=[1 0 0; 0 1 0; 0 0 1]
  Rigid Transform (Orientation) : sm_lib/Frames and Transforms/Rigid Transform  TranslationMethod=None  TranslationStandardOffset=0  TranslationLengthUnit=m  TranslationStandardAxis=+Z  TranslationCartesianOffset=constraint.loc  TranslationROffset=0  TranslationROffsetUnits=m  TranslationZOffset=0  TranslationZOffsetUnits=m  TranslationThetaOffset=0  TranslationThetaOffsetUnits=deg  RotationMethod=RotationMatrix  RotationAngleUnits=rad  RotationStandardAxis=+Y  RotationAngle=0  RotationArbitraryAxis=[0 1 0]  FollAlignAxisA=+X  BaseAlignAxisA=+Y  FollAlignAxisB=+Y  BaseAlignAxisB=+Z  RotationSequenceAxes=FollowerAxes  RotationSequence=XYX  RotationSequenceAngles=[0 0 0]  RotationSequenceAnglesUnits=deg  RotationMatrix=constraint.orientation.rotationMatrix
  Rigid Transform (Orientation)1 : sm_lib/Frames and Transforms/Rigid Transform  TranslationMethod=None  TranslationStandardOffset=0  TranslationLengthUnit=m  TranslationStandardAxis=+Z  TranslationCartesianOffset=constraint.loc  TranslationROffset=0  TranslationROffsetUnits=m  TranslationZOffset=0  TranslationZOffsetUnits=m  TranslationThetaOffset=0  TranslationThetaOffsetUnits=deg  RotationMethod=RotationMatrix  RotationAngleUnits=rad  RotationStandardAxis=+Y  RotationAngle=0  RotationArbitraryAxis=[0 1 0]  FollAlignAxisA=+X  BaseAlignAxisA=+Y  FollAlignAxisB=+Y  BaseAlignAxisB=+Z  RotationSequenceAxes=FollowerAxes  RotationSequence=XYX  RotationSequenceAngles=[0 0 0]  RotationSequenceAnglesUnits=deg  RotationMatrix=constraint.orientation.rotationMatrix
  Selector : Selector  InputPortWidth=3  IndexOptions=Index vector (dialog)  Indices=[1 3 2]  OutputSizes=1
  Selector1 : Selector  InputPortWidth=3  IndexOptions=Index vector (dialog)  Indices=[2]  OutputSizes=1
  Selector2 : Selector  InputPortWidth=3  IndexOptions=Index vector (dialog)  Indices=[1 3 2]  OutputSizes=1
  Selector3 : Selector  InputPortWidth=3  IndexOptions=Index vector (dialog)  Indices=[2]  OutputSizes=1
  output : ToWorkspace  VariableName=constraint11_out  SaveFormat=Structure With Time  SampleTime=-1
  F : PMIOPort  Port=1  Side=Right
  B : PMIOPort  Port=2  Side=Left
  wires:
  Assignment4/1 -> Mux/2
  PS-Simulink Converter4/1 -> Selector2/1
  Gain4/1 -> Assignment4/2
  Selector3/1 -> Gain4/1
  Selector2/1 -> Assignment4/1, Selector3/1
  Assignment3/1 -> Mux/1
  Gain3/1 -> Assignment3/2
  Selector1/1 -> Gain3/1
  Selector/1 -> Selector1/1, Assignment3/1
  PS-Simulink Converter3/1 -> Selector/1
  Mux3/1 -> Assignment1/2
  Mux4/1 -> Assignment/2
  Constant/1 -> Assignment/1
  Constant1/1 -> Assignment1/1
  Constant2/1 -> Assignment2/1
  Assignment2/1 -> Mux1/3  "acceleration"
  Assignment1/1 -> Mux1/2  "velocity"
  Assignment/1 -> Mux1/1  "position"
  Mux/1 -> Mux1/4  "Constraint Forces"
  Mux1/1 -> output/1
  PS-Simulink Converter5/1 -> Gain5/1
  Gain5/1 -> Mux2/2
  PS-Simulink Converter6/1 -> Mux2/3
  PS-Simulink Converter7/1 -> Mux2/1
  Mux2/1 -> Assignment2/2
  PS-Simulink Converter2/1 -> Gain2/1
  Gain2/1 -> Mux3/2
  PS-Simulink Converter8/1 -> Mux3/3
  PS-Simulink Converter9/1 -> Mux3/1
  PS-Simulink Converter11/1 -> Gain1/1
  Gain1/1 -> Mux4/2
  PS-Simulink Converter1/1 -> Mux4/1
  PS-Simulink Converter10/1 -> Mux4/3
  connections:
  Rigid Transform (Position)1/LConn1 -- F/RConn1
  Rigid Transform (Position)1/RConn1 -- Rigid Transform (Orientation)1/LConn1
  Rigid Transform (Orientation)1/RConn1 -- Rigid Transform (90 X)1/LConn1
  Rigid Transform (Orientation)/RConn1 -- Rigid Transform (90 X)/LConn1
  Rigid Transform (Position)/RConn1 -- Rigid Transform (Orientation)/LConn1
  Rigid Transform (Position)/LConn1 -- B/RConn1
  PS-Simulink Converter4/LConn1 -- CONSTRAINT (Gimbal Joint)/RConn12
  PS-Simulink Converter3/LConn1 -- CONSTRAINT (Gimbal Joint)/RConn11
  PS-Simulink Converter5/LConn1 -- CONSTRAINT (Gimbal Joint)/RConn10
  PS-Simulink Converter6/LConn1 -- CONSTRAINT (Gimbal Joint)/RConn7
  PS-Simulink Converter7/LConn1 -- CONSTRAINT (Gimbal Joint)/RConn4
  CONSTRAINT (Gimbal Joint)/LConn1 -- Rigid Transform (90 X)/RConn1
  PS-Simulink Converter2/LConn1 -- CONSTRAINT (Gimbal Joint)/RConn9
  CONSTRAINT (Gimbal Joint)/RConn6 -- PS-Simulink Converter8/LConn1
  PS-Simulink Converter9/LConn1 -- CONSTRAINT (Gimbal Joint)/RConn3
  CONSTRAINT (Gimbal Joint)/RConn2 -- PS-Simulink Converter1/LConn1
  CONSTRAINT (Gimbal Joint)/RConn5 -- PS-Simulink Converter10/LConn1
  PS-Simulink Converter11/LConn1 -- CONSTRAINT (Gimbal Joint)/RConn8
  Rigid Transform (90 X)1/RConn1 -- CONSTRAINT (Gimbal Joint)/RConn1

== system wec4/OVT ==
  vref_x : Inport
  vref_z : Inport  Port=2
  ekfFreqZ : Inport  Port=3
  ekfFreqX : Inport  Port=4
  Rel. vel X : Inport  Port=5
  Rel. vel. Z : Inport  Port=6
  Anti wind-up controller 1 : Subsystem
  Anti wind-up controller 2 : Subsystem
  Clock1 : Clock
  Divide4 : Product  Inputs=**
  Divide5 : Product  Inputs=**
  Product11 : Product
  Product3 : Product
  Ramp gain2 : Lookup_n-D  NumberOfTableDimensions=1  BreakpointsForDimension1=arControllerRampTime  Table=arControllerRampGain  InternalRulePriority=Speed  RndMeth=Simplest
  Selector1 : Selector  InputPortWidth=6  IndexOptions=Index vector (dialog)  Indices=3  OutputSizes=1
  Selector18 : Selector  InputPortWidth=6  IndexOptions=Index vector (dialog)  Indices=1  OutputSizes=1
  Selector2 : Selector  InputPortWidth=6  IndexOptions=Index vector (dialog)  Indices=3  OutputSizes=1
  Selector3 : Selector  InputPortWidth=6  IndexOptions=Index vector (dialog)  Indices=1  OutputSizes=1
  Sum{1,5..6,11} (4 alike) : Sum  Inputs=|+-
  Trnasformation X-Z into PTO forces : Subsystem
  adaptiveLaw1 : Lookup_n-D  NumberOfTableDimensions=1  BreakpointsForDimension1=arFrequencyRange  Table=arFrequencyRange./arFrequencyRange  InternalRulePriority=Speed  RndMeth=Simplest
  adaptiveLaw2 : Lookup_n-D  NumberOfTableDimensions=1  BreakpointsForDimension1=arFrequencyRange  Table=arFrequencyRange./arFrequencyRange  InternalRulePriority=Speed  RndMeth=Simplest
  forceDemand1 : Outport
  forceDemand2 : Outport  Port=2
  forceDemand3 : Outport  Port=3
  forceDemand4 : Outport  Port=4
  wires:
  Divide5/1 -> Sum1/1
  Sum1/1 -> Anti wind-up controller 1/1(error)
  Divide4/1 -> Sum11/1
  Sum11/1 -> Anti wind-up controller 2/1(error)
  adaptiveLaw2/1 -> Divide4/2
  vref_x/1 -> Divide4/1
  ekfFreqX/1 -> adaptiveLaw2/1
  adaptiveLaw1/1 -> Divide5/1
  ekfFreqZ/1 -> adaptiveLaw1/1
  vref_z/1 -> Divide5/2
  [vel1] -> Selector1/1, Selector18/1
  [vel2] -> Selector2/1, Selector3/1
  Selector18/1 -> Sum5/1
  Selector3/1 -> Sum5/2
  Selector1/1 -> Sum6/1
  Selector2/1 -> Sum6/2
  Anti wind-up controller 2/1(forceDemand1) -> Trnasformation X-Z into PTO forces/1(Force X)  "Force X"
  Anti wind-up controller 1/1(forceDemand1) -> Trnasformation X-Z into PTO forces/2(Force Z)  "Force Z"
  Clock1/1 -> Ramp gain2/1
  Ramp gain2/1 -> Product3/1, Product11/2
  Product3/1 -> forceDemand2/1, forceDemand1/1  "F1"
  Trnasformation X-Z into PTO forces/1(Force PTOs 3-4) -> Product11/1
  Product11/1 -> forceDemand4/1, forceDemand3/1
  Trnasformation X-Z into PTO forces/2(Force PTOs 1-2) -> Product3/2
  Rel. vel X/1 -> Sum11/2
  Rel. vel. Z/1 -> Sum1/2

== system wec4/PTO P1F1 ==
  P1F1_force : Inport
  Demux : Demux  Outputs=3
  PTO P1F1 visu : Subsystem  AncestorBlock=WECSim_Lib/Body Elements/Rigid Body  Variant=on
  Scope1 : Scope
  Selector1 : Selector  InputPortWidth=6  IndexOptions=Index vector (dialog)  Indices=3  OutputSizes=1
  Selector2 : Selector  InputPortWidth=6  IndexOptions=Index vector (dialog)  Indices=3  OutputSizes=1
  Selector3 : Selector  InputPortWidth=6  IndexOptions=Index vector (dialog)  Indices=3  OutputSizes=1
  SideTether1_preload : Constant  Value=SidePTO1Preload
  Sum : Sum  Inputs=++|
  Terminator : Terminator
  Translational PTO Actuation Force P1F1 : Subsystem  AncestorBlock=WECSim_Lib/PTOs/Translational PTO Actuation Force
  F : PMIOPort  Port=1  Side=Right
  B : PMIOPort  Port=2  Side=Left
  P1F1_response : Outport
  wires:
  SideTether1_preload/1 -> Sum/1
  P1F1_force/1 -> Sum/2
  Sum/1 -> Translational PTO Actuation Force P1F1/1(Force)
  Translational PTO Actuation Force P1F1/1(Response) -> P1F1_response/1, Demux/1
  Translational PTO Actuation Force P1F1/2(ptoForce) -> Selector2/1
  Demux/1 -> Selector3/1
  Demux/2 -> Scope1/1, Selector1/1
  Selector3/1 -> [ptoDis1]
  Selector2/1 -> [ptoForce1]
  Demux/3 -> Terminator/1
  Selector1/1 -> [ptoSpd1]
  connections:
  Translational PTO Actuation Force P1F1/LConn1 -- B/RConn1
  F/RConn1 -- Translational PTO Actuation Force P1F1/RConn1 -- PTO P1F1 visu/RConn1

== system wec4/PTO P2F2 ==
  P2F2_force : Inport
  Demux : Demux  Outputs=3
  PTO P2F2 visu : Subsystem  AncestorBlock=WECSim_Lib/Body Elements/Rigid Body  Variant=on
  Scope1 : Scope
  Scope2 : Scope
  Selector1 : Selector  InputPortWidth=6  IndexOptions=Index vector (dialog)  Indices=3  OutputSizes=1
  Selector2 : Selector  InputPortWidth=6  IndexOptions=Index vector (dialog)  Indices=3  OutputSizes=1
  Selector3 : Selector  InputPortWidth=6  IndexOptions=Index vector (dialog)  Indices=3  OutputSizes=1
  SideTether2_preload : Constant  Value=SidePTO2Preload
  Sum : Sum  Inputs=++|
  Terminator : Terminator
  Translational PTO Actuation Force P2F2 : Subsystem  AncestorBlock=WECSim_Lib/PTOs/Translational PTO Actuation Force
  F : PMIOPort  Port=1  Side=Right
  B : PMIOPort  Port=2  Side=Left
  P2F2_response : Outport
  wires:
  SideTether2_preload/1 -> Sum/1
  P2F2_force/1 -> Sum/2
  Sum/1 -> Translational PTO Actuation Force P2F2/1(Force)
  Translational PTO Actuation Force P2F2/1(Response) -> Demux/1, P2F2_response/1
  Demux/1 -> Scope2/1, Selector3/1
  Demux/2 -> Scope1/1, Selector1/1
  Selector3/1 -> [ptoDis2]
  Selector1/1 -> [ptoSpd2]
  Selector2/1 -> [ptoForce2]
  Demux/3 -> Terminator/1
  Translational PTO Actuation Force P2F2/2(ptoForce) -> Selector2/1
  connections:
  Translational PTO Actuation Force P2F2/LConn1 -- B/RConn1
  Translational PTO Actuation Force P2F2/RConn1 -- PTO P2F2 visu/RConn1 -- F/RConn1

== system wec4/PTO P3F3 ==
  P3F3_force : Inport
  Demux : Demux  Outputs=3
  PTO P3F3 visu : Subsystem  AncestorBlock=WECSim_Lib/Body Elements/Rigid Body  Variant=on
  Scope1 : Scope
  Scope2 : Scope
  Selector1 : Selector  InputPortWidth=6  IndexOptions=Index vector (dialog)  Indices=3  OutputSizes=1
  Selector2 : Selector  InputPortWidth=6  IndexOptions=Index vector (dialog)  Indices=3  OutputSizes=1
  Selector3 : Selector  InputPortWidth=6  IndexOptions=Index vector (dialog)  Indices=3  OutputSizes=1
  SideTether3_preload : Constant  Value=SidePTO3Preload
  Sum : Sum  Inputs=++|
  Terminator : Terminator
  Translational PTO Actuation Force P3F3 : Subsystem  AncestorBlock=WECSim_Lib/PTOs/Translational PTO Actuation Force
  F : PMIOPort  Port=1  Side=Right
  B : PMIOPort  Port=2  Side=Left
  P3F3_response : Outport
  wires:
  SideTether3_preload/1 -> Sum/1
  P3F3_force/1 -> Sum/2
  Sum/1 -> Translational PTO Actuation Force P3F3/1(Force)
  Translational PTO Actuation Force P3F3/1(Response) -> Demux/1, P3F3_response/1
  Demux/1 -> Scope2/1, Selector3/1
  Demux/2 -> Scope1/1, Selector1/1
  Selector3/1 -> [ptoDis3]
  Selector1/1 -> [ptoSpd3]
  Selector2/1 -> [ptoForce3]
  Demux/3 -> Terminator/1
  Translational PTO Actuation Force P3F3/2(ptoForce) -> Selector2/1
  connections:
  Translational PTO Actuation Force P3F3/LConn1 -- B/RConn1
  F/RConn1 -- PTO P3F3 visu/RConn1 -- Translational PTO Actuation Force P3F3/RConn1

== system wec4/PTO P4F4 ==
  P4F4_force : Inport
  Demux : Demux  Outputs=3
  PTO P4F4 visu : Subsystem  AncestorBlock=WECSim_Lib/Body Elements/Rigid Body  Variant=on
  Scope1 : Scope
  Scope2 : Scope
  Selector1 : Selector  InputPortWidth=6  IndexOptions=Index vector (dialog)  Indices=3  OutputSizes=1
  Selector2 : Selector  InputPortWidth=6  IndexOptions=Index vector (dialog)  Indices=3  OutputSizes=1
  Selector3 : Selector  InputPortWidth=6  IndexOptions=Index vector (dialog)  Indices=3  OutputSizes=1
  SideTether4_preload : Constant  Value=SidePTO4Preload
  Sum : Sum  Inputs=++|
  Terminator : Terminator
  Translational PTO Actuation Force P4F4 : Subsystem  AncestorBlock=WECSim_Lib/PTOs/Translational PTO Actuation Force
  F : PMIOPort  Port=1  Side=Right
  B : PMIOPort  Port=2  Side=Left
  P4F4_response : Outport
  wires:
  SideTether4_preload/1 -> Sum/1
  P4F4_force/1 -> Sum/2
  Sum/1 -> Translational PTO Actuation Force P4F4/1(Force)
  Translational PTO Actuation Force P4F4/1(Response) -> Demux/1, P4F4_response/1
  Demux/1 -> Scope2/1, Selector3/1
  Demux/2 -> Scope1/1, Selector1/1
  Selector3/1 -> [ptoDis4]
  Selector1/1 -> [ptoSpd4]
  Selector2/1 -> [ptoForce4]
  Demux/3 -> Terminator/1
  Translational PTO Actuation Force P4F4/2(ptoForce) -> Selector2/1
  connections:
  Translational PTO Actuation Force P4F4/RConn1 -- PTO P4F4 visu/RConn1 -- F/RConn1
  Translational PTO Actuation Force P4F4/LConn1 -- B/RConn1

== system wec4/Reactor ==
  note: 1) Add Subsystem or Model blocks as valid variant choices. 2) You cannot connect blocks at this level. At simulation, connectivity is automatically determined, based on the active variant and port name matching.
  Hydrodynamic Body : Subsystem  VariantControl=sv_b2_hydroBody
  Non-Hydro Body : Subsystem  VariantControl=sv_b2_nonHydroBody
  Conn : PMIOPort  Port=1  Side=Right
